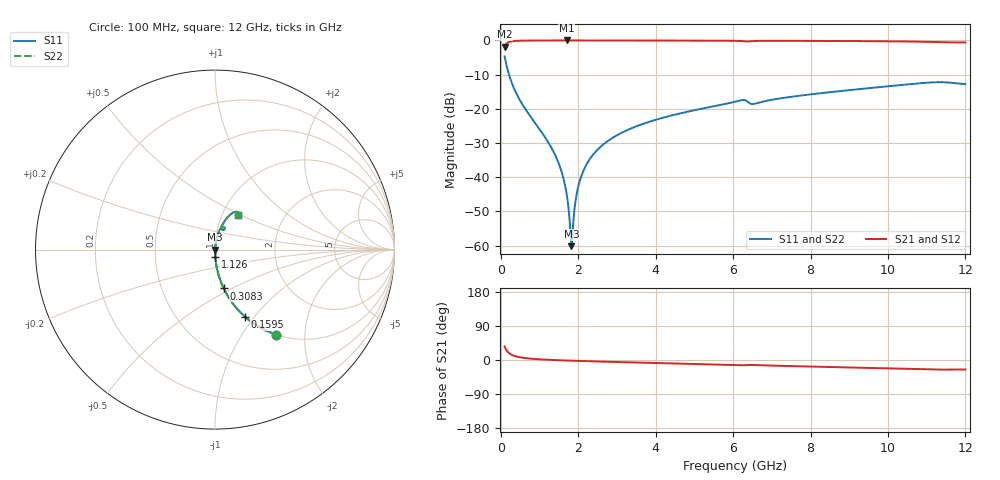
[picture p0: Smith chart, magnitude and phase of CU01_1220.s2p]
! S-parameter model data by Modelithics Inc. support@modelithics.com 813-866-6335 Tampa FL USA
! S-Parameter data specifications:
! Substrate: 20-mil Rogers, substrate thickness, H=0.508mm, Dielectric constant, Er=3.75
! PCB Mounting Pad Footprint: Pad width, PadW=0.35mm , Pad length, PadL=0.30mm , Pad gap, PadG (edge-to-edge)=0.25mm , Reference planes=0.85mm apart
! Created Tue May  8 14:01:25 2018
# hz S ma R 50
! 2 Port Network Data from SP1.SP block
! freq  magS11  angS11  magS21  angS21  magS12  angS12  magS22  angS22
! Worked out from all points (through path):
!   801 points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, 100 MHz to 12 GHz, reference 50 ohm
!   highest |S21| = -0.01 dB at 1.706 GHz (marker M1); lowest = -1.8 dB at 100 MHz (marker M2)
!   group delay of S21, straight-line fit = 7.62 ps
!   lowest |S11| = -60.2 dB at 1.825 GHz (marker M3), VSWR 1.00, Z = 50.1 - j0.0124 ohm
!   |S11| at or under -10 dB: 213.7 MHz to end of sweep
!   |S22| runs from -60.2 to -4.7 dB; largest |S21 - S12| = 0
!   S11 on the Smith chart (normalised r, x): 100 MHz: 1.00, -1.44; 159.5 MHz: 1.00, -0.90; 308.2 MHz: 1.00, -0.45; 1.126 GHz: 1.00, -0.08; 12 GHz: 1.19, +0.48
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1e8  0.5842 -54.3  0.8112 35.6  0.8112 35.6  0.5842 -54.3
1.595e8  0.4098 -65.9  0.9118 24.0  0.9118 24.0  0.4098 -65.9
3.0825e8  0.2219 -77.4  0.9746 12.5  0.9746 12.5  0.2219 -77.4
5.76e8  0.1122 -83.8  0.9931 5.9  0.9931 5.9  0.1122 -83.8
1.126375e9  0.03975 -87.7  0.9984 1.2  0.9984 1.2  0.03975 -87.7
1.49825e9  0.01585 -87.3  0.999 -0.6  0.999 -0.6  0.01585 -87.3
1.61725e9  0.009743 -85.6  0.999 -1.1  0.999 -1.1  0.009743 -85.6
1.7065e9  0.005513 -81.5  0.999 -1.4  0.999 -1.4  0.005513 -81.5
1.780875e9  0.002268 -66.5  0.999 -1.7  0.999 -1.7  0.002268 -66.5
1.8255e9  0.0009803 -7.3  0.999 -1.8  0.999 -1.8  0.0009803 -7.3
1.870125e9  0.002069 59.6  0.999 -2.0  0.999 -2.0  0.002069 59.6
1.97425e9  0.006198 78.3  0.9989 -2.3  0.9989 -2.3  0.006198 78.3
2.09325e9  0.01083 81.8  0.9989 -2.7  0.9989 -2.7  0.01083 81.8
2.346125e9  0.02003 83.4  0.9987 -3.5  0.9987 -3.5  0.02003 83.4
2.732875e9  0.0328 83.4  0.9983 -4.6  0.9983 -4.6  0.0328 83.4
3.298125e9  0.0497 82.4  0.9974 -6.1  0.9974 -6.1  0.0497 82.4
4.071625e9  0.07096 80.7  0.996 -8.1  0.996 -8.1  0.07096 80.7
6.05e9  0.1269 74.4  0.9867 -13.3  0.9867 -13.3  0.1269 74.4
6.526e9  0.1178 70.0  0.979 -13.2  0.979 -13.2  0.1178 70.0
8.04325e9  0.1636 71.7  0.9838 -17.4  0.9838 -17.4  0.1636 71.7
1.002162e10  0.2142 66.2  0.9711 -22.3  0.9711 -22.3  0.2142 66.2
1.2e10  0.2303 56.0  0.9376 -25.1  0.9376 -25.1  0.2303 56.0
